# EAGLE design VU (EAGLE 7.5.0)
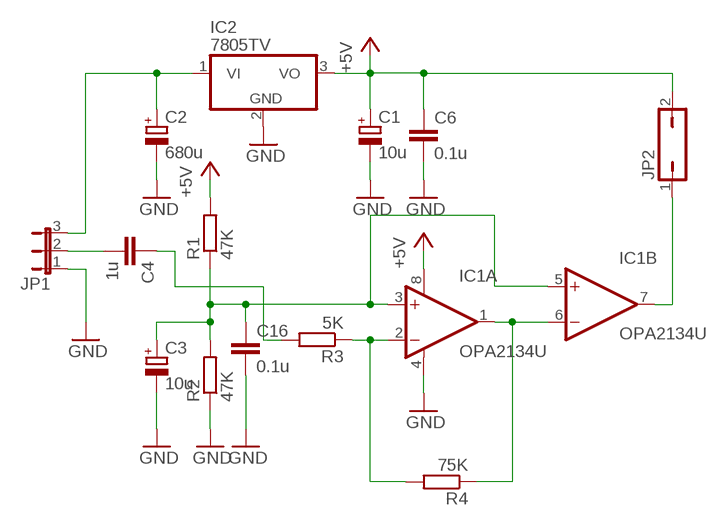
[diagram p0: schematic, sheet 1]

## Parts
C1  10u  CPOL-EUE2.5-6  [E2,5-6]
C2  680u  CPOL-EUE3.5-8  [E3,5-8]
C3  10u  CPOL-EUCT6032  [CT6032]
C4  1u  C-EUC1206  [C1206]
C6  0.1u  C-EUC1206  [C1206]
C16  0.1u  C-EUC1206  [C1206]
IC1  OPA2134U  [SO08]
IC2  7805TV  [TO220V]
JP1  JP2E  [JP2]
JP2  JP1Q  [JP1]
R1  47K  R-EU_R0805  [R0805]
R2  47K  R-EU_R0805  [R0805]
R3  5K  R-EU_R0805  [R0805]
R4  75K  R-EU_R0805  [R0805]

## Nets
+5V: C1.+ C6.1 IC1.8(A:V+) IC2.3(VO) JP2.2 R1.2
GND: C1.- C2.- C3.- C6.2 C16.2 IC1.4(A:V-) IC2.2(GND) JP1.1 R2.1
N$1: C3.+ C16.1 IC1.3(A:+IN) IC1.5(B:+IN) R1.1 R2.2
N$2: IC1.2(A:-IN) R3.1 R4.2
N$3: C4.1 R3.2
N$4: C2.+ IC2.1(VI) JP1.3
N$6: C4.2 JP1.2
N$8: IC1.1(A:OUT) IC1.6(B:-IN) R4.1
N$10: IC1.7(B:OUT) JP2.1

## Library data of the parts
C1-C3 = rcl:CPOL-EU: POLARIZED CAPACITOR, European symbol
C4 C6 C16 = rcl:C-EU: CAPACITOR, European symbol
IC1 = burr-brown:OPA2134: Operational Amplifier; MF: TEXAS INSTRUMENTS; MPN: OPA2134UA; OC_FARNELL: 1206935; OC_NEWARK: 35C1847
IC2 = linear:78*: Positive VOLTAGE REGULATOR Source: http://cache.national.com/ds/LM/LM78L05.pdf http://www.fairchildsemi.com/ds/LM/LM7805.pdf
JP1 = jumper:JP2E: JUMPER
JP2 = jumper:JP1Q: JUMPER
R1-R4 = rcl:R-EU_: RESISTOR, European symbol

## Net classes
0 default: width 0.152 mm, drill 0.61 mm, clearance 0.152 mm

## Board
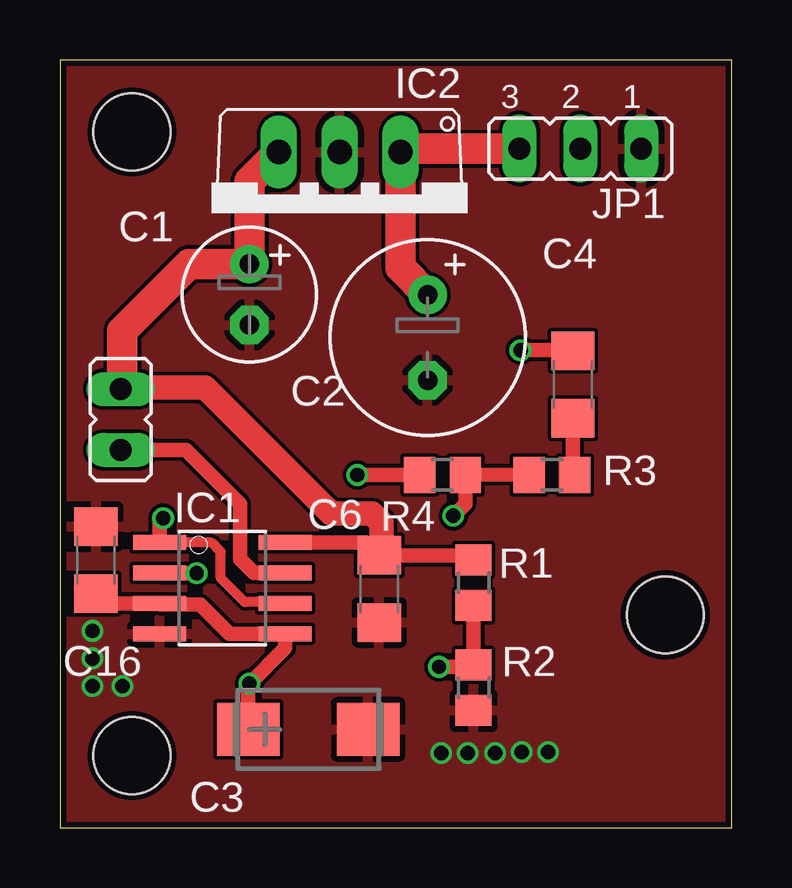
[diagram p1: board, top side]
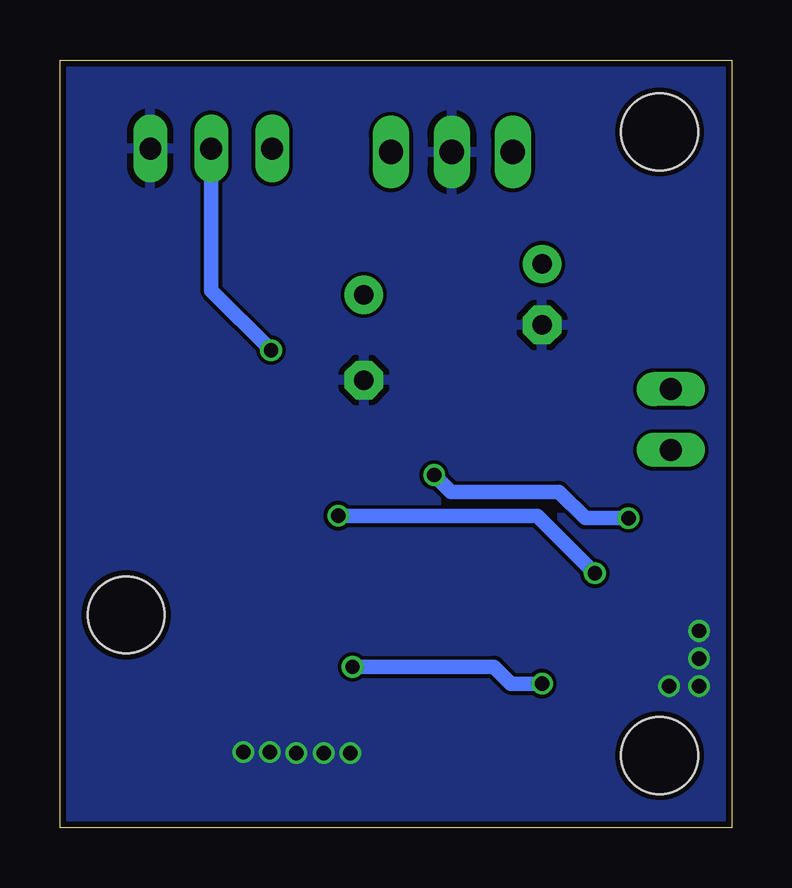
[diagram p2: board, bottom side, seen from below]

Size 28 x 32 mm. Coordinates in mm from the lower left corner, seen from the top.
Outline: 0,0 28,0 28,32 0,32 0,0
Copper layers (1*16): Top 0.035mm / dielectric 1.5mm / Bottom 0.035mm
Design rules "ITEADstudio_DRC": minimum track width 6mil, minimum drill 12mil, track to track 6mil, track to pad 6mil, pad to pad 6mil, via to via 6mil, smd to smd 0mil, copper to edge 10mil, drill to drill 10mil, minimum pad ring 10mil, minimum via ring 6mil, stop-mask expansion 2mil, vias tented up to drill 100mil, thermal gap 10mil
Holes 3.2 mm at 3,3 3,29 25.24,8.86

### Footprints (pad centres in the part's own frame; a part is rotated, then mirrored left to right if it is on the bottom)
E2,5-6 = drill 0.813 pad 1.6: + -1.27,0 | drill 0.813 pad 1.6 octagon: - 1.27,0
E3,5-8 = drill 0.813 pad 1.6: + -1.778,0 | drill 0.813 pad 1.6 octagon: - 1.778,0
CT6032 = smd 2.6 x 2.2: + -2.5,0; - 2.5,0
C1206 = smd 1.6 x 1.8: 1 -1.4,0; 2 1.4,0
SO08 = smd 0.61 x 2.21: 1 -1.905,-2.616; 2 -0.635,-2.616; 3 0.635,-2.616; 4 1.905,-2.616; 5 1.905,2.616; 6 0.635,2.616; 7 -0.635,2.616; 8 -1.905,2.616
TO220V = drill 1.016 long: 1 -2.54,-2.54; 2 0,-2.54; 3 2.54,-2.54
JP2 = drill 0.914 long: 1 -2.54,0; 2 0,0; 3 2.54,0
JP1 = drill 0.914 long: 1 0,-1.27; 2 0,1.27
R0805 = smd 1.3 x 1.5: 1 -0.95,0; 2 0.95,0

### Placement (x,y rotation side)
C1  7.9,22.22 270 top
C2  15.33,20.43 270 top
C3  10.35,4.09 0 top
C4  21.39,18.47 90 top
C6  13.31,9.95 270 top
C16  1.5,11.15 90 top
IC1  6.77,9.98 270 top
IC2  11.66,25.62 180 top
JP1  21.69,28.31 180 top
JP2  2.53,17.01 0 top
R1  17.24,10.21 90 top
R2  17.24,5.83 90 top
R3  20.51,14.7 0 top
R4  15.95,14.7 0 top

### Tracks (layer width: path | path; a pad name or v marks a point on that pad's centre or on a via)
+5V
  Top 0.61: IC1.8 12.78,11.88 C6.1 17.05,11.35 R1.2 17.13,11.35
  Top 1.016: 2.6,18.35 6.05,18.35 11.3,13.1 13,13.1 13.4,12.7 13.4,11.44 C6.1
  Top 1.27: IC2.3 7.9,26.94 C1.+ 5.39,23.49 2.6,20.7 2.6,18.35 JP2.2
GND  (via drill 0.6)
  other vias: 2.6,5.9 1.35,8.2 1.35,7.05 1.35,5.9 15.9,3.1 17,3.1 18.15,3.1 19.25,3.15 20.35,3.15
  pour Top: -0.8,34.1 29.35,34.1 29.35,-1.5 -0.8,-1.5
  pour Bottom: -1.1,34.35 30,34.1 30,-1.8 -1.1,-1.55
N$1  (via drill 0.6)
  Top 0.61: R1.1 R2.2 17.16,6.7 v15.8,6.7 | C3.+ 7.85,5.95 v7.9,6 9.39,7.49 IC1.5 7.08,8.07 5.85,9.3 4.2,9.3 IC1.3 1.91,9.35 C16.1
  Bottom 0.61: v15.8,6.7 9.9,6.7 9.2,6 v7.9,6
N$2  (via drill 0.6)
  Top 0.61: R3.1 16.95,14.71 R4.2 16.9,13.5 v16.4,13 | IC1.2 4.17,10.6 v5.7,10.6
  Bottom 0.61: v16.4,13 8.1,13 v5.7,10.6
N$3
  Top 0.61: C4.1 21.39,14.78 R3.2
N$4
  Top 1.27: C2.+ 14.2,23.34 IC2.1 14.35,28.31 JP1.3
N$6  (via drill 0.6)
  Top 0.61: v19.2,19.9 21.36,19.9 C4.2
  Bottom 0.61: JP1.2 21.69,22.39 v19.2,19.9
N$8  (via drill 0.6)
  Top 0.406: IC1.6 9.33,9.4 7.7,9.4 6.7,10.4 6.7,11.5 6.32,11.88 IC1.1
  Top 0.61: R4.1 v12.4,14.7 | v4.3,12.9 4.15,12.75 IC1.1
  Bottom 0.61: v12.4,14.7 11.7,14 7.2,14 6.1,12.9 v4.3,12.9
N$10
  Top 0.61: IC1.7 8.09,10.62 7.5,11.2 7.5,13.5 5.26,15.74 JP2.1 2.96,15.74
